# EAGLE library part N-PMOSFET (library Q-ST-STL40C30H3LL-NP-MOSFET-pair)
http://www.digikey.com/product-detail/en/stmicroelectronics/STL40C30H3LL/497-15314-1-ND/5170833
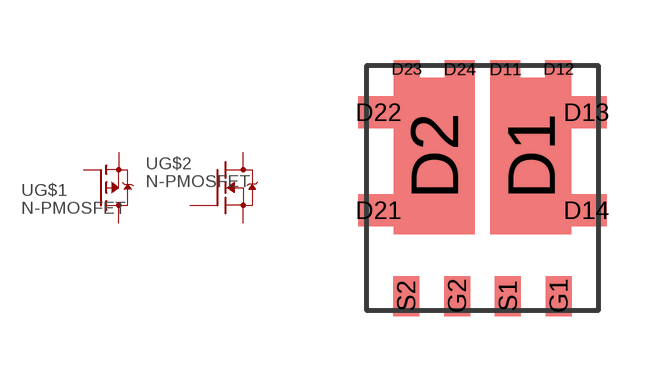
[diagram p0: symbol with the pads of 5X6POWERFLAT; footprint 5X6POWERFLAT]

Designator prefix -; gates G$1=P-MOSFET G$2=N-MOSFET-GDS-D

## N-PMOSFET  [5X6POWERFLAT]
D1  G$1:D  pas
D2  G$2:D  pas
D11  G$1:D  pas
D12  G$1:D  pas
D13  G$1:D  pas
D14  G$1:D  pas
D21  G$2:D  pas
D22  G$2:D  pas
D23  G$2:D  pas
D24  G$2:D  pas
G1  G$1:G  pas
G2  G$2:G  pas
S1  G$1:S  pas
S2  G$2:S  pas

## Footprint 5X6POWERFLAT (pad centres in mm)
smd 2.025 x 3.9: D1 1.21,1.95; D2 -1.21,1.95
smd 0.75 x 0.45: D11 0.572,4.125; D24 -0.572,4.125
smd 0.65 x 0.45: D12 1.898,4.125; D23 -1.898,4.125
smd 1 x 0.8: D13 2.6,3.04; D14 2.6,0.59; D21 -2.6,0.59; D22 -2.6,3.04
smd 0.65 x 1: G1 1.905,-1.55; G2 -0.635,-1.55; S1 0.635,-1.55; S2 -1.905,-1.55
